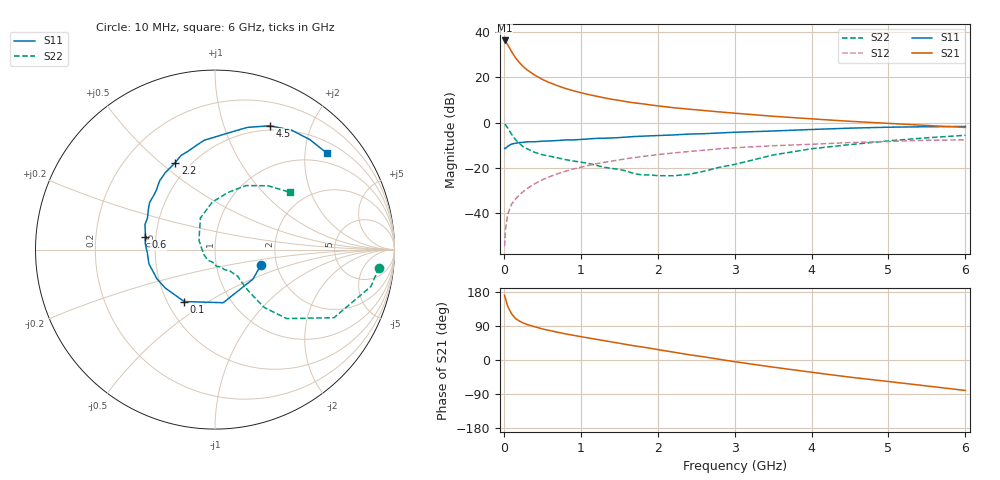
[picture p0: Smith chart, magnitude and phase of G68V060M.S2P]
! SIEMENS Small Signal Semiconductors
! BFG193
! Si NPN RF Bipolar Junction Transistor in SOT223
! VCE = 8 V  IC = 60 mA
! Common Emitter S-Parameters:  August  1996
# GHz  S  MA  R  50
!  f  S11  S21  S12  S22
! GHz  MAG  ANG  MAG  ANG  MAG  ANG  MAG  ANG
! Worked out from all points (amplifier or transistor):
!   36 points, 10 MHz to 6 GHz, reference 50 ohm
!   highest |S21| = 36.2 dB at 10 MHz (marker M1)
!   |S21| within 3 dB of that: start of sweep to 69.05 MHz
!   unconditionally stable (mu >= 1): 446.4 MHz to 2.381 GHz
!   at 250 MHz: K = 0.92, MSG = 27.6 dB, |S12| = -30.5 dB
!   at 1.4 GHz: K = 1.04, MAG = 12.3 dB, |S12| = -17.0 dB
!   at 6 GHz: K = 0.89, MSG = 2.7 dB, |S12| = -7.6 dB
!   S11 on the Smith chart (normalised r, x): 10 MHz: 1.65, -0.31; 100 MHz: 0.61, -0.40; 600 MHz: 0.44, +0.07; 2.2 GHz: 0.41, +0.56; 4.5 GHz: 0.45, +1.44; 6 GHz: 0.75, +2.49
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0.01  0.2694 -18.9  64.26 170.5  0.0019 92.0  0.9192 -6.3
0.02  0.268 -37.7  61.71 163.0  0.0042 77.7  0.8927 -13.3
0.05  0.2995 -81.2  51.98 141.9  0.0096 71.7  0.7636 -29.8
0.1  0.3365 -120.7  36.65 122.2  0.0159 67.9  0.5541 -43.9
0.15  0.3501 -142.2  26.87 109.8  0.0206 65.9  0.4229 -49.6
0.2  0.362 -153.2  21.16 103.0  0.0254 68.6  0.3501 -50.4
0.25  0.3672 -161.6  17.25 97.8  0.0299 68.4  0.2959 -51.0
0.3  0.3764 -167.7  14.57 93.8  0.0352 69.8  0.266 -51.1
0.4  0.3775 -177.0  11.12 87.8  0.0448 69.6  0.2218 -50.3
0.5  0.3895 175.3  8.92 82.0  0.0548 68.9  0.1961 -49.6
0.6  0.394 169.9  7.498 77.6  0.0649 67.8  0.1814 -50.6
0.8  0.4146 160.2  5.645 69.1  0.0845 64.5  0.153 -54.0
0.9  0.4147 155.3  5.037 65.2  0.0948 62.9  0.1428 -55.3
1.1  0.4357 148.3  4.146 58.2  0.1138 59.4  0.1258 -63.9
1.3  0.4517 141.6  3.522 51.2  0.1333 55.3  0.1043 -70.7
1.6  0.4809 131.2  2.869 40.6  0.1609 48.7  0.085 -90.0
2.2  0.5332 114.5  2.13 21.0  0.2139 35.1  0.0674 -151.6
2.8  0.5904 100.0  1.719 1.9  0.2643 21.2  0.1034 149.7
3.5  0.6526 83.8  1.377 -18.8  0.309 4.0  0.1934 114.9
4.5  0.754 66.2  1.066 -45.3  0.3634 -15.9  0.3271 77.0
5.5  0.8093 49.2  0.864 -68.5  0.4094 -39.2  0.4627 50.2
6  0.8226 40.9  0.781 -80.4  0.4156 -52.6  0.5249 37.5
